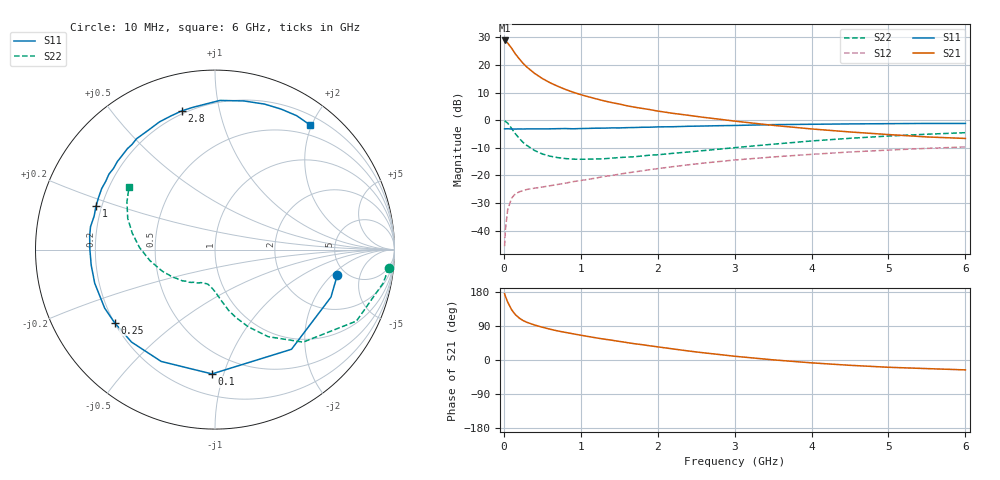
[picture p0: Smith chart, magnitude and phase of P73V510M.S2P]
! SIEMENS Small Signal Semiconductors
! BFP196
! Si NPN RF Bipolar Junction Transistor in SOT143
! VCE = 3.5 V  IC = 10 mA
! Common Emitter S-Parameters:  May  1996
# GHz  S  MA  R  50
!  f  S11  S21  S12  S22
! GHz  MAG  ANG  MAG  ANG  MAG  ANG  MAG  ANG
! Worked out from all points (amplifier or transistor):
!   36 points, 10 MHz to 6 GHz, reference 50 ohm
!   highest |S21| = 28.9 dB at 10 MHz (marker M1)
!   |S21| within 3 dB of that: start of sweep to 105.6 MHz
!   unconditionally stable (mu >= 1): 871.4 MHz to 3.273 GHz
!   at 250 MHz: K = 0.40, MSG = 23.1 dB, |S12| = -25.5 dB
!   at 1.4 GHz: K = 1.14, MAG = 11.0 dB, |S12| = -20.1 dB
!   at 6 GHz: K = 0.97, MSG = 1.5 dB, |S12| = -9.7 dB
!   S11 on the Smith chart (normalised r, x): 10 MHz: 4.27, -2.32; 100 MHz: 0.34, -0.92; 250 MHz: 0.20, -0.31; 1 GHz: 0.18, +0.17; 2.8 GHz: 0.18, +0.77; 6 GHz: 0.34, +1.98
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0.01  0.6963 -11.6  27.91 175.0  0.0052 84.2  0.9745 -5.9
0.02  0.6982 -22.3  27.16 168.2  0.0103 79.1  0.9552 -11.3
0.05  0.7 -52.5  25.04 152.9  0.0238 66.7  0.8829 -26.8
0.1  0.6929 -91.4  20.3 133.0  0.0385 51.2  0.7119 -46.4
0.15  0.6915 -115.7  15.91 119.7  0.0462 41.8  0.5683 -58.6
0.2  0.6941 -132.1  13 110.7  0.0502 37.3  0.4682 -66.7
0.25  0.6921 -144.0  10.76 104.1  0.053 34.3  0.3953 -72.9
0.3  0.6959 -152.0  9.169 99.4  0.0555 33.5  0.3481 -77.3
0.4  0.6958 -164.4  7.063 92.3  0.0585 32.6  0.2825 -83.4
0.5  0.6951 -172.8  5.698 86.5  0.0615 34.0  0.2443 -88.2
0.6  0.6972 179.9  4.783 81.3  0.0648 35.1  0.2228 -92.5
0.7  0.7023 173.9  4.128 76.7  0.0684 36.6  0.2099 -96.0
0.8  0.7052 169.6  3.616 72.9  0.0722 37.8  0.2016 -99.4
1  0.7058 159.9  2.908 65.4  0.0806 40.6  0.1958 -104.6
1.1  0.7107 155.9  2.656 61.9  0.0849 41.5  0.1969 -107.5
1.6  0.7327 137.9  1.827 46.0  0.1105 43.9  0.2142 -121.0
2.2  0.7615 119.4  1.331 29.2  0.1438 42.3  0.251 -136.0
2.8  0.7951 103.3  1.043 14.5  0.1781 37.8  0.2984 -152.9
3.5  0.8316 88.1  0.807 0.4  0.2155 30.6  0.3672 -170.3
4.5  0.8564 71.2  0.612 -14.0  0.2654 19.7  0.4697 168.8
5.5  0.8739 58.6  0.497 -22.7  0.3084 8.3  0.5573 151.7
6  0.8733 52.6  0.467 -26.1  0.3278 2.1  0.5936 143.8
